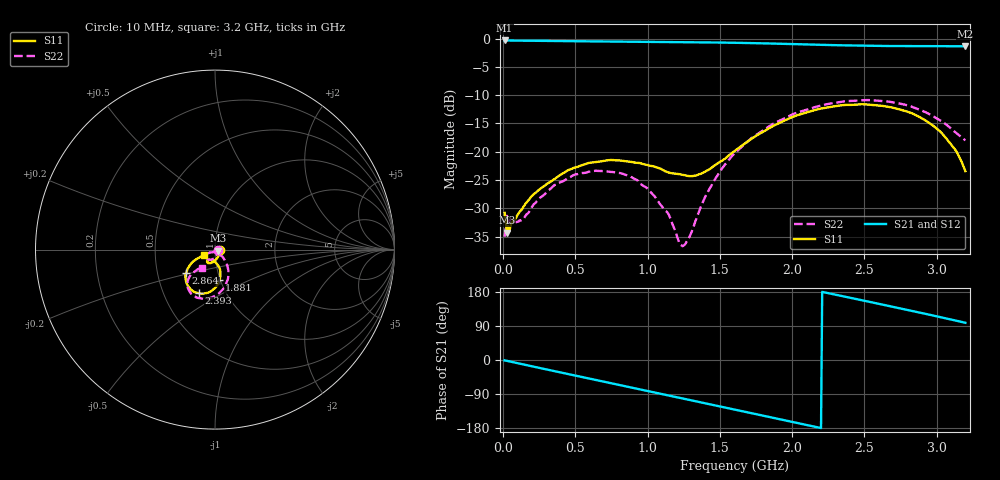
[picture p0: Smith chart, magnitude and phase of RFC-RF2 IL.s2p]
!Agilent Technologies,N5230A,MY45001650,A.07.50.48
!Agilent N5230A: A.07.50.48
!Date: Monday, December 05, 2022 16:04:11
!Correction: S11(Full 2 Port(1,2))
!S21(Full 2 Port(1,2))
!S12(Full 2 Port(1,2))
!S22(Full 2 Port(1,2))
!S2P File: Measurements: S11, S21, S12, S22:
# Hz S  dB  R 50
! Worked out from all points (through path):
!   400 points, 10 MHz to 3.2 GHz, reference 50 ohm
!   highest |S21| = -0.33 dB at 10 MHz (marker M1); lowest = -1.4 dB at 3.2 GHz (marker M2)
!   group delay of S21, straight-line fit = 226 ps
!   lowest |S11| = -34.3 dB at 25.99 MHz (marker M3), VSWR 1.04, Z = 51.9 - j0.663 ohm
!   |S11| at or under -10 dB: start of sweep to end of sweep
!   |S22| runs from -36.7 to -10.9 dB; largest |S21 - S12| = 0.0011
!   S11 on the Smith chart (normalised r, x): 10 MHz: 1.06, -0.00; 1.881 GHz: 0.99, -0.35; 2.393 GHz: 0.75, -0.39; 2.864 GHz: 0.70, -0.19; 3.2 GHz: 0.89, -0.06
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1e7  -30.80 -3.9  -0.33 -0.9  -0.34 -0.9  -35.01 -2.3
2.598997e7  -34.29 -19.3  -0.35 -2.1  -0.35 -2.1  -31.33 -11.5
3.398496e7  -33.14 -18.5  -0.34 -2.9  -0.34 -2.9  -32.56 -15.3
4.197995e7  -34.12 -20.8  -0.35 -3.5  -0.35 -3.5  -32.58 -16.8
1.059398e8  -30.93 -40.2  -0.37 -8.9  -0.37 -8.9  -32.36 -43.3
2.178697e8  -27.37 -66.3  -0.39 -18.2  -0.39 -18.2  -29.16 -79.7
3.537845e8  -24.84 -87.3  -0.43 -29.3  -0.43 -29.3  -25.91 -96.9
5.456642e8  -22.37 -105.0  -0.48 -45.0  -0.48 -45.0  -23.76 -118.2
8.654637e8  -21.73 -122.6  -0.56 -70.8  -0.56 -70.8  -24.22 -142.4
1.081328e9  -22.91 -122.5  -0.60 -88.2  -0.60 -88.2  -29.10 -151.4
1.145288e9  -23.67 -121.2  -0.61 -93.4  -0.61 -93.4  -31.03 -145.0
1.225238e9  -23.98 -112.6  -0.62 -99.8  -0.62 -99.8  -36.39 -114.2
1.249223e9  -24.11 -110.1  -0.63 -101.8  -0.63 -101.8  -36.59 -99.3
1.425113e9  -23.15 -88.4  -0.67 -116.2  -0.68 -116.2  -26.71 -46.1
1.608997e9  -19.72 -76.6  -0.74 -131.2  -0.75 -131.2  -20.13 -49.7
1.880827e9  -15.30 -81.7  -0.89 -153.6  -0.89 -153.5  -14.91 -66.5
2.136667e9  -12.78 -94.5  -1.06 -174.4  -1.06 -174.4  -12.28 -84.5
2.392506e9  -11.72 -110.5  -1.22 165.0  -1.21 165.0  -11.03 -101.9
2.672331e9  -12.09 -128.5  -1.32 142.5  -1.31 142.5  -11.16 -119.9
2.864211e9  -13.63 -140.8  -1.33 126.8  -1.33 126.8  -12.39 -129.7
3.0401e9  -16.82 -151.0  -1.34 112.0  -1.33 112.0  -14.70 -134.0
3.2e9  -23.43 -151.9  -1.37 98.2  -1.37 98.2  -17.99 -125.2
